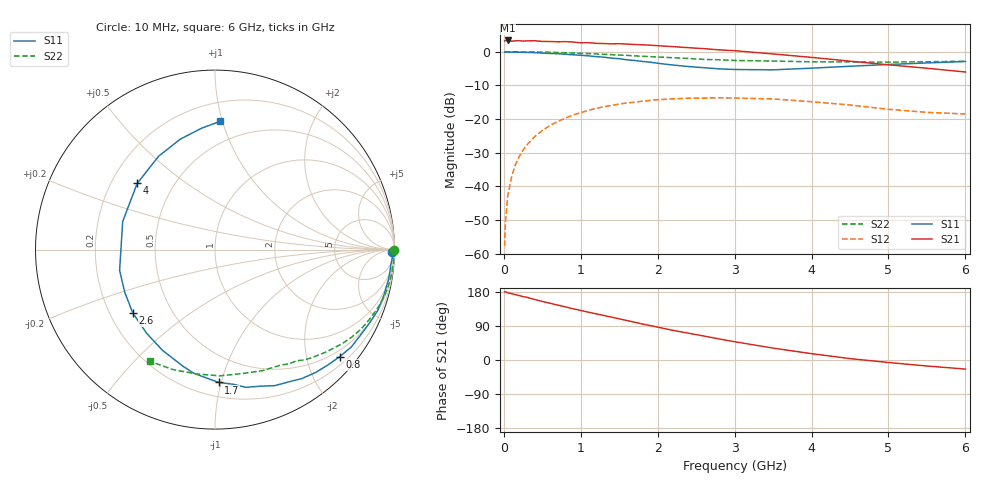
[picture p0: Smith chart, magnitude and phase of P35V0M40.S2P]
! SIEMENS Small Signal Semiconductors
! BFP181
! Si NPN RF Bipolar Junction Transistor in SOT143
! VCE = 5 V  IC = 0.4 mA
! Common Emitter S-Parameters:  March  1996
# GHz  S  MA  R  50
!  f  S11  S21  S12  S22
! GHz  MAG  ANG  MAG  ANG  MAG  ANG  MAG  ANG
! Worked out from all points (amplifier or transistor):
!   36 points, 10 MHz to 6 GHz, reference 50 ohm
!   highest |S21| = 3.3 dB at 50 MHz (marker M1)
!   |S21| within 3 dB of that: start of sweep to 2.968 GHz
!   unconditionally stable (mu >= 1): 3.902 GHz to end of sweep
!   at 250 MHz: K = 0.08, MSG = 16.2 dB, |S12| = -29.2 dB
!   at 1.4 GHz: K = 0.42, MSG = 9.1 dB, |S12| = -15.9 dB
!   at 6 GHz: K = 1.49, MAG = 2.1 dB, |S12| = -18.5 dB
!   S11 on the Smith chart (normalised r, x): 10 MHz: 71, -66; 800 MHz: 0.36, -2.65; 1.7 GHz: 0.30, -0.98; 2.6 GHz: 0.30, -0.31; 4 GHz: 0.31, +0.34; 6 GHz: 0.34, +0.98
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0.01  0.985 -0.8  1.442 179.7  0.0013 79.3  0.9989 -0.2
0.02  0.9872 -0.9  1.458 179.9  0.0029 85.2  0.9982 -0.5
0.05  0.9899 -2.2  1.467 177.6  0.0072 91.4  0.9982 -1.3
0.1  0.9828 -5.2  1.433 175.0  0.0138 85.2  0.9978 -2.5
0.15  0.9822 -7.8  1.449 172.5  0.021 84.2  0.9974 -3.7
0.25  0.9762 -12.8  1.436 167.3  0.0347 80.5  0.9935 -6.3
0.4  0.9686 -20.3  1.453 159.7  0.0547 75.3  0.9905 -10.0
0.5  0.9532 -25.4  1.421 154.5  0.0676 71.3  0.9847 -12.4
0.8  0.9154 -40.7  1.409 140.1  0.1033 60.5  0.9639 -19.6
1.1  0.8666 -56.0  1.36 126.0  0.1346 50.1  0.9351 -26.4
1.5  0.7863 -77.4  1.314 108.6  0.1669 37.4  0.8909 -34.7
1.7  0.7403 -88.4  1.279 99.7  0.1784 31.4  0.8663 -38.6
1.9  0.6989 -99.8  1.25 91.0  0.189 25.8  0.8443 -42.2
2.2  0.633 -117.5  1.188 78.2  0.1994 17.9  0.8128 -47.4
2.6  0.5781 -142.5  1.109 63.3  0.2046 8.5  0.7682 -53.8
3  0.544 -167.7  1.034 48.2  0.2047 -0.9  0.7404 -60.3
3.5  0.5376 163.1  0.925 31.4  0.1988 -10.4  0.725 -68.3
4  0.5692 139.6  0.823 16.7  0.181 -18.0  0.7072 -77.6
4.5  0.6077 121.1  0.723 3.7  0.1616 -23.8  0.7039 -87.9
5  0.6451 107.4  0.638 -6.6  0.1396 -25.1  0.7002 -98.5
5.5  0.6805 96.3  0.568 -15.9  0.1257 -22.1  0.7084 -109.3
6  0.7157 87.6  0.499 -23.9  0.119 -17.3  0.7208 -120.4
